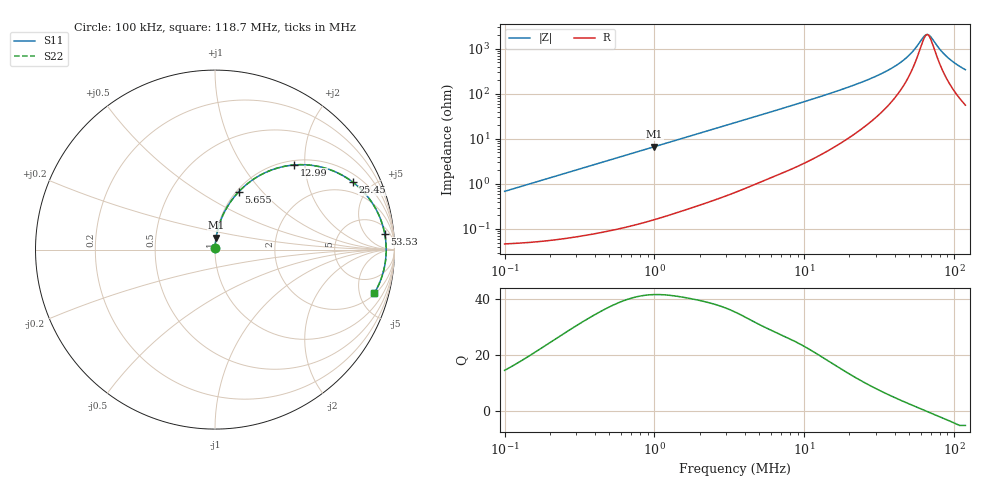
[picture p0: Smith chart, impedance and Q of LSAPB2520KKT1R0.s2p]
! LSAPB2520KKT1R0  S-PARAMETER MODEL  ( General Type )
! Model Generated by TAIYO YUDEN Corporation (http://www.ty-top.com)
! Version 2.0
! TAIYO YUDEN Control No. 20210629
! Copyright(c) 2015 TAIYO YUDEN CO.,LTD. All Rights Reserved.
! Product Description (link to TY-COMPAS)
! https://ds.yuden.co.jp/TYCOMPAS/or/detail?pn=LSAPB2520KKT1R0M&u=M
! Products Name : Inductors
! Characteristics :
!  Inductance : 1.0 uH , SRF(min) : -Hz , DC Resistance(max) : 0.053 Ohm
!  Rated Current : Saturation :3800 mA , Temp Rise : 3000 mA (40 degC)
!  Case Size : 2.5 x 2.0 / 0.098 x 0.079 [mm/inch] , Thickness : 1 / 0.039 [mm/inch]
!  (Conditions: Temperature = 25 degC , DC Bias Current/Voltage = 0A / 0V)
! External Node Assignments :
!  1  o---GGG---o  2
! GND o---------o GND
! Frequency Range : 0.1MHz  -  118.695536MHz  [ 402 STEP ]
# MHz S RI R 50
! Freq[MHz].  S11 Real  S11 Imag  S21 Real  S21 Imag  S12 Real  S12 Imag  S22 Real  S22 Imag
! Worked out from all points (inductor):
!   401 points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, 100 kHz to 118.7 MHz, reference 50 ohm
!   read as one part in series: L = 1.09 uH near 103.6 kHz
!   highest Q = 41.7 at 998.1 kHz (marker M1), where L = 1.07 uH
!   self-resonance near 65.99 MHz
!   S11 on the Smith chart (normalised r, x): 100 kHz: 1.00, +0.01; 5.655 MHz: 1.03, +0.75; 12.99 MHz: 1.09, +1.76; 25.45 MHz: 1.38, +3.87; 53.53 MHz: 9, +16; 118.7 MHz: 2.12, -6.75
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0.1  0.000513 0.00682  0.9995 -0.00682  0.9995 -0.00682  0.000513 0.00682
0.327316  0.00119 0.0222  0.9988 -0.0222  0.9988 -0.0222  0.00119 0.0222
0.998139  0.00607 0.0666  0.9939 -0.0666  0.9939 -0.0666  0.00607 0.0666
1.07136  0.00685 0.0714  0.9931 -0.0714  0.9931 -0.0714  0.00685 0.0714
1.990437  0.0205 0.1297  0.9795 -0.1297  0.9795 -0.1297  0.0205 0.1297
3.445222  0.0553 0.2148  0.9447 -0.2148  0.9447 -0.2148  0.0553 0.2148
5.654935  0.1316 0.3215  0.8684 -0.3215  0.8684 -0.3215  0.1316 0.3215
8.056554  0.2319 0.4031  0.7681 -0.4031  0.7681 -0.4031  0.2319 0.4031
11.27678  0.3715 0.4606  0.6285 -0.4606  0.6285 -0.4606  0.3715 0.4606
12.99193  0.441 0.4716  0.559 -0.4716  0.559 -0.4716  0.441 0.4716
17.86583  0.6055 0.4564  0.3945 -0.4564  0.3945 -0.4564  0.6055 0.4564
25.45335  0.7692 0.3749  0.2308 -0.3749  0.2308 -0.3749  0.7692 0.3749
36.91074  0.8877 0.2412  0.1123 -0.2412  0.1123 -0.2412  0.8877 0.2412
45.64422  0.9278 0.1548  0.0722 -0.1548  0.0722 -0.1548  0.9278 0.1548
53.52547  0.9456 0.0883  0.0544 -0.0883  0.0544 -0.0883  0.9456 0.0883
62.76757  0.9535 0.0212  0.0465 -0.0212  0.0465 -0.0212  0.9535 0.0212
65.02906  0.954 0.00621  0.046 -0.00621  0.046 -0.00621  0.954 0.00621
67.37203  0.9539 -0.00874  0.0461 0.00874  0.0461 0.00874  0.9539 -0.00874
81.85149  0.9454 -0.0909  0.0546 0.0909  0.0546 0.0909  0.9454 -0.0909
89.4246  0.9367 -0.128  0.0633 0.128  0.0633 0.128  0.9367 -0.128
103.0257  0.9161 -0.1868  0.0839 0.1868  0.0839 0.1868  0.9161 -0.1868
118.6955  0.887 -0.2441  0.113 0.2441  0.113 0.2441  0.887 -0.2441
